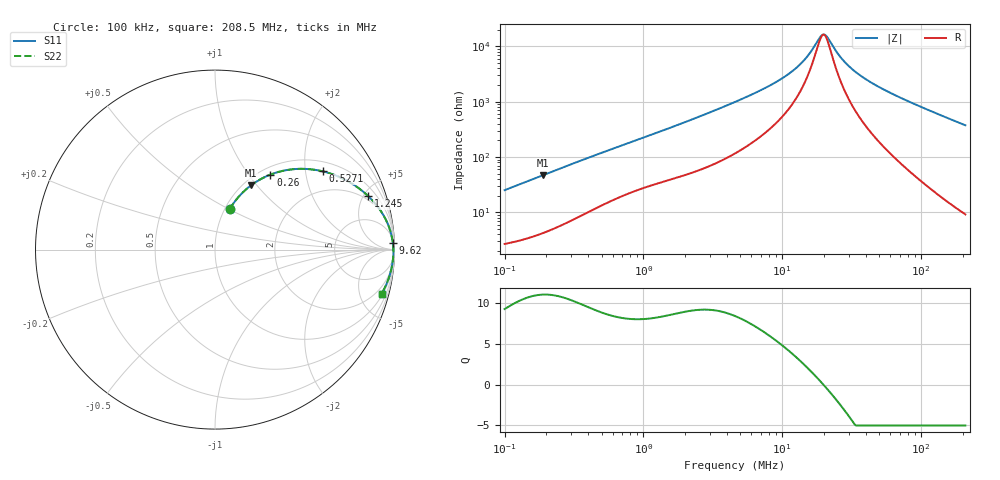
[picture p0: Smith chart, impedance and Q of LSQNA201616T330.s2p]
! LSQNA201616T330  S-PARAMETER MODEL  ( General Type )
! Model Generated by TAIYO YUDEN Corporation (http://www.ty-top.com)
! Version 2.0
! TAIYO YUDEN Control No. 100810NF25SB-FKC
! Copyright(c) 2007 TAIYO YUDEN CO.,LTD. All Rights Reserved.
! Product Description (link to TY-COMPAS)
! https://ds.yuden.co.jp/TYCOMPAS/or/detail?pn=LSQNA201616T330K&u=M
! Products Name : Inductors
! Characteristics :
!  Inductance : 33 uH , SRF(min) : 14 MHz , DC Resistance(max) : 2.21 Ohm
!  Rated Current : Saturation :130 mA , Temp Rise : 270 mA (40 degC)
!  Case Size : 2.0 x 1.6 / 0.079 x 0.063 [mm/inch] , Thickness : 1.6 / 0.063 [mm/inch]
!  (Conditions: Temperature = 25 degC , DC Bias Current/Voltage = 0A / 0V)
! External Node Assignments :
!  1  o---GGG---o  2
! GND o---------o GND
! Frequency Range : 0.1MHz  -  208.503118MHz  [ 402 STEP ]
# MHz S RI R 50
! Freq[MHz].  S11 Real  S11 Imag  S21 Real  S21 Imag  S12 Real  S12 Imag  S22 Real  S22 Imag
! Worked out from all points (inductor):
!   401 points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, 100 kHz to 208.5 MHz, reference 50 ohm
!   read as one part in series: L = 39.8 uH near 103.9 kHz
!   highest Q = 11.1 at 187.9 kHz (marker M1), where L = 39.5 uH
!   self-resonance near 19.51 MHz
!   S11 on the Smith chart (normalised r, x): 100 kHz: 1.05, +0.50; 259.9 kHz: 1.12, +1.28; 527.1 kHz: 1.28, +2.49; 1.245 MHz: 1.66, +5.44; 9.62 MHz: 11, +49; 208.5 MHz: 1.18, -7.48
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0.1  0.0812 0.2247  0.9188 -0.2247  0.9188 -0.2247  0.0812 0.2247
0.187857  0.2006 0.3579  0.7994 -0.3579  0.7994 -0.3579  0.2006 0.3579
0.25995  0.3082 0.4176  0.6918 -0.4176  0.6918 -0.4176  0.3082 0.4176
0.359709  0.4405 0.4483  0.5595 -0.4483  0.5595 -0.4483  0.4405 0.4483
0.527117  0.5998 0.4361  0.4002 -0.4361  0.4002 -0.4361  0.5998 0.4361
0.802524  0.7461 0.3778  0.2539 -0.3778  0.2539 -0.3778  0.7461 0.3778
1.245395  0.855 0.2967  0.145 -0.2967  0.145 -0.2967  0.855 0.2967
1.293906  0.8624 0.2895  0.1376 -0.2895  0.1376 -0.2895  0.8624 0.2895
2.295283  0.9411 0.187  0.0589 -0.187  0.0589 -0.187  0.9411 0.187
4.654297  0.9791 0.0954  0.0209 -0.0954  0.0209 -0.0954  0.9791 0.0954
9.619882  0.9908 0.0388  0.00925 -0.0388  0.00925 -0.0388  0.9908 0.0388
13.05973  0.9927 0.0214  0.00731 -0.0214  0.00731 -0.0214  0.9927 0.0214
16.42508  0.9935 0.00946  0.00646 -0.00946  0.00646 -0.00946  0.9935 0.00946
18.77552  0.9938 0.00271  0.00617 -0.00271  0.00617 -0.00271  0.9938 0.00271
20.26671  0.9939 -0.00113  0.00606 0.00113  0.00606 0.00113  0.9939 -0.00113
21.46232  0.994 -0.00402  0.00601 0.00402  0.00601 0.00402  0.994 -0.00402
26.48208  0.994 -0.0148  0.00601 0.0148  0.00601 0.0148  0.994 -0.0148
31.45084  0.9937 -0.0242  0.00626 0.0242  0.00626 0.0242  0.9937 -0.0242
41.09615  0.9928 -0.0402  0.00719 0.0402  0.00719 0.0402  0.9928 -0.0402
59.08252  0.99 -0.0667  0.01 0.0667  0.01 0.0667  0.99 -0.0667
113.1315  0.9749 -0.1375  0.0251 0.1375  0.0251 0.1375  0.9749 -0.1375
208.5031  0.928 -0.2465  0.072 0.2465  0.072 0.2465  0.928 -0.2465
